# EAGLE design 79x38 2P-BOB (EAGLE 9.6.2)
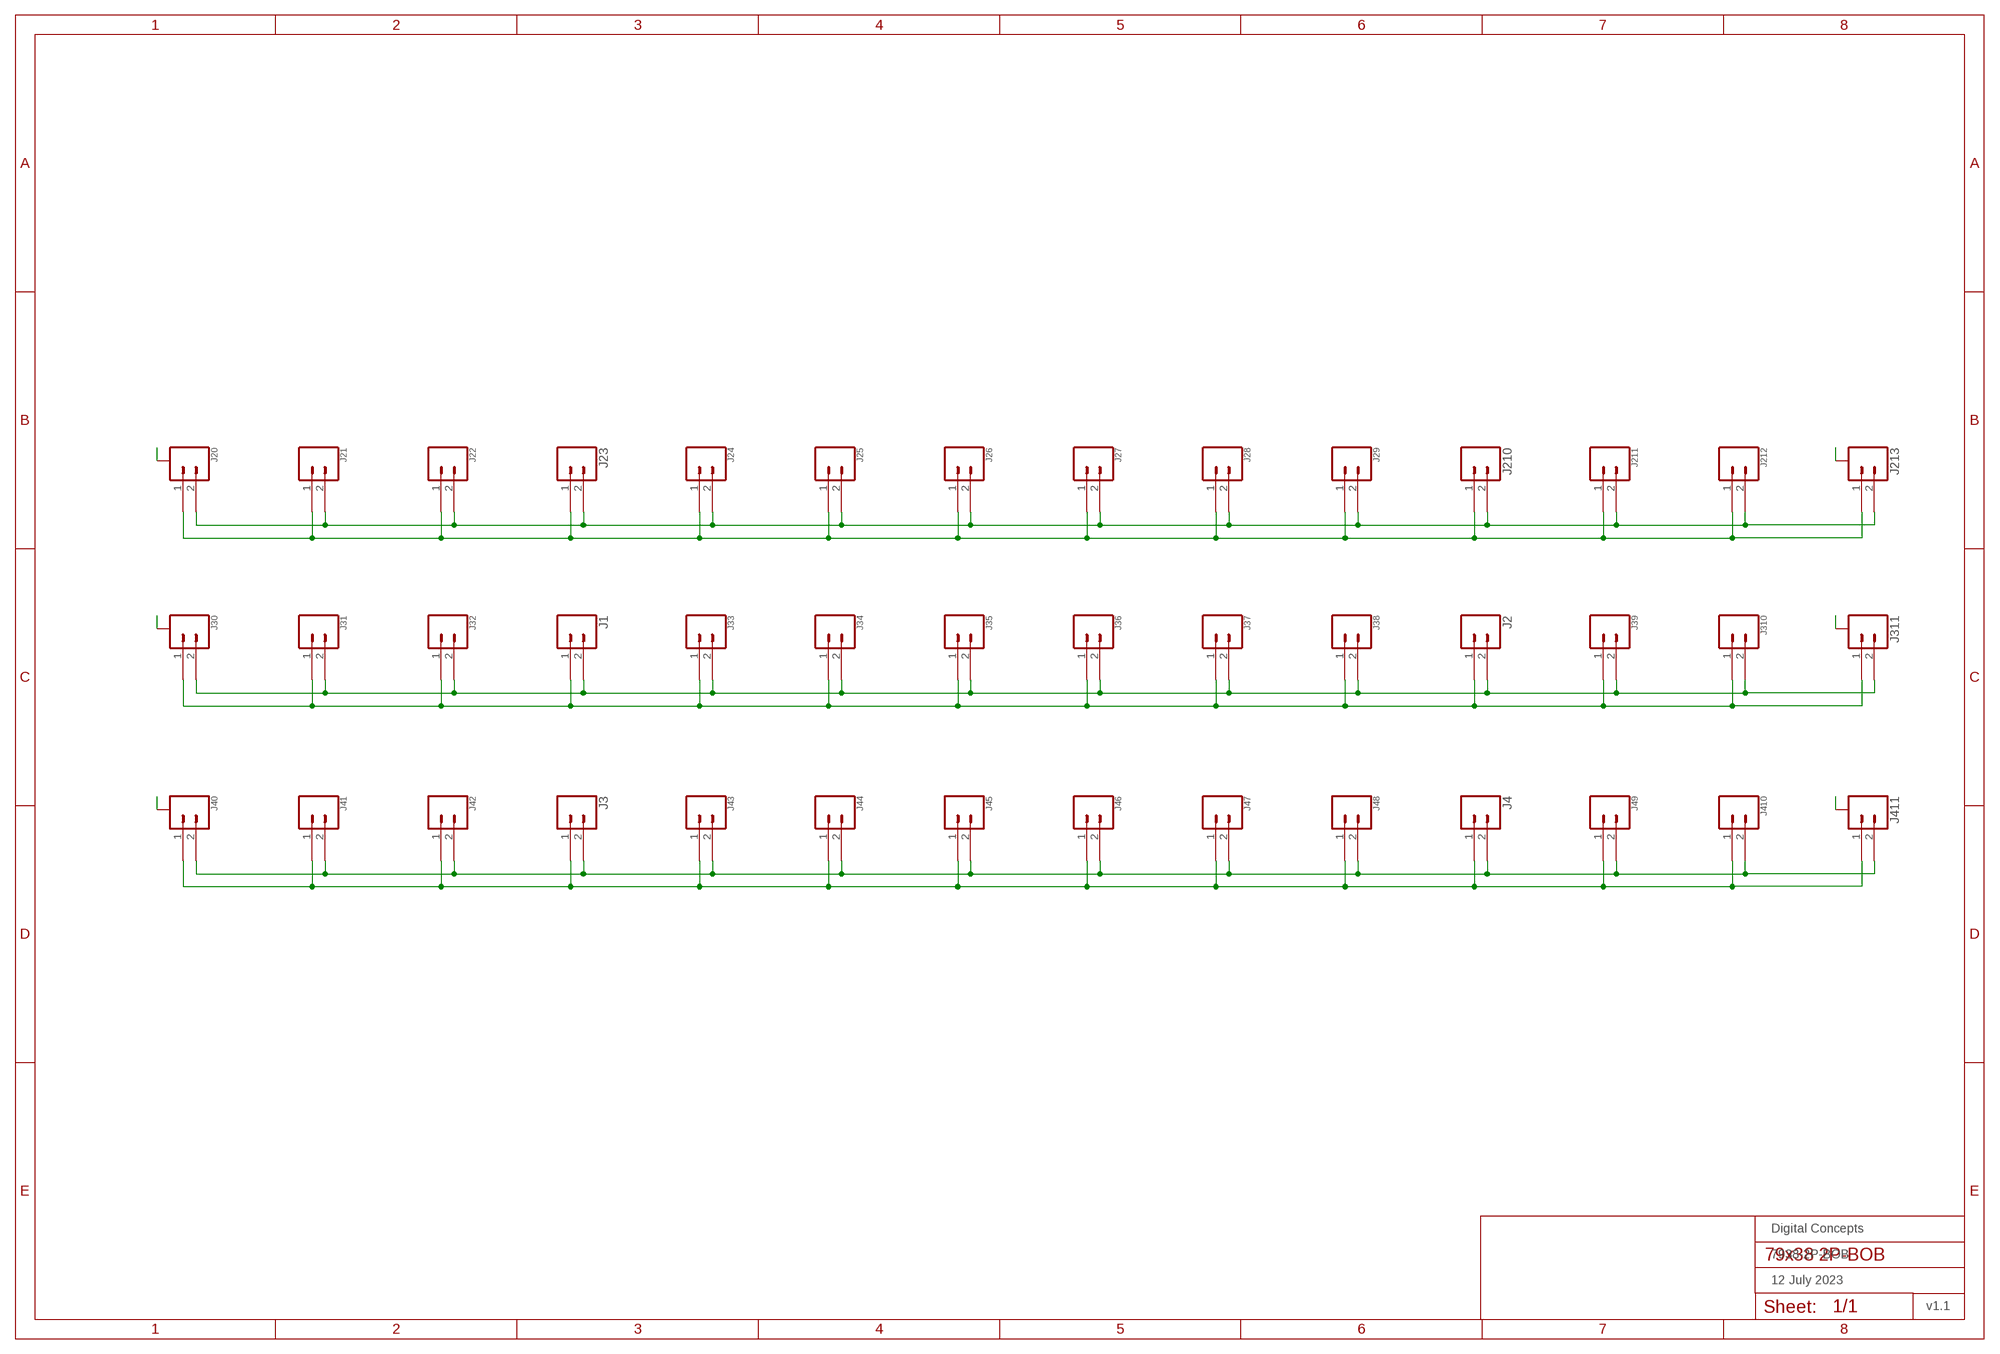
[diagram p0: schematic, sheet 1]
FRAME1 (FRAME-A3L-LOC): DATE: 12 July 2023; OWNER: Digital Concepts; TITLE: 7938-2P-BOB; VERSION: v1.1

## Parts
J1  JST-XH2.54-2-VERTICAL  [JST-XH2.4-2-VERTICAL]
J2  JST-XH2.54-2-VERTICAL  [JST-XH2.4-2-VERTICAL]
J3  JST-XH2.54-2-VERTICAL  [JST-XH2.4-2-VERTICAL]
J4  JST-XH2.54-2-VERTICAL  [JST-XH2.4-2-VERTICAL]
J20  JST-SH1.0-2-SMD-VERTICAL  [JST-SH1.0-2-VERTICAL]
J21  JST-GH1.25-2-VERTICAL  [JST-GH1.25-2-VERTICAL]
J22  JST-PH2.0-2-VERTICAL  [JST-PH2.0-2-VERTICAL]
J23  JST-XH2.54-2-VERTICAL  [JST-XH2.4-2-VERTICAL]
J24  HEADER-1X2-GENERIC  [CONN_02-GENERIC]
J25  HEADER-1X2-GENERIC  [CONN_02-GENERIC]
J26  HEADER-1X2-GENERIC  [CONN_02-GENERIC]
J27  HEADER-1X2-GENERIC  [CONN_02-GENERIC]
J28  HEADER-1X2-GENERIC  [CONN_02-GENERIC]
J29  HEADER-1X2-GENERIC  [CONN_02-GENERIC]
J30  JST-SH1.0-2-SMD-VERTICAL  [JST-SH1.0-2-VERTICAL]
J31  JST-GH1.25-2-VERTICAL  [JST-GH1.25-2-VERTICAL]
J32  JST-PH2.0-2-VERTICAL  [JST-PH2.0-2-VERTICAL]
J33  HEADER-1X2-GENERIC  [CONN_02-GENERIC]
J34  HEADER-1X2-GENERIC  [CONN_02-GENERIC]
J35  HEADER-1X2-GENERIC  [CONN_02-GENERIC]
J36  HEADER-1X2-GENERIC  [CONN_02-GENERIC]
J37  HEADER-1X2-GENERIC  [CONN_02-GENERIC]
J38  HEADER-1X2-GENERIC  [CONN_02-GENERIC]
J39  JST-PH2.0-2-VERTICAL  [JST-PH2.0-2-VERTICAL]
J40  JST-SH1.0-2-SMD-VERTICAL  [JST-SH1.0-2-VERTICAL]
J41  JST-GH1.25-2-VERTICAL  [JST-GH1.25-2-VERTICAL]
J42  JST-PH2.0-2-VERTICAL  [JST-PH2.0-2-VERTICAL]
J43  HEADER-1X2-GENERIC  [CONN_02-GENERIC]
J44  HEADER-1X2-GENERIC  [CONN_02-GENERIC]
J45  HEADER-1X2-GENERIC  [CONN_02-GENERIC]
J46  HEADER-1X2-GENERIC  [CONN_02-GENERIC]
J47  HEADER-1X2-GENERIC  [CONN_02-GENERIC]
J48  HEADER-1X2-GENERIC  [CONN_02-GENERIC]
J49  JST-PH2.0-2-VERTICAL  [JST-PH2.0-2-VERTICAL]
J210  JST-XH2.54-2-VERTICAL  [JST-XH2.4-2-VERTICAL]
J211  JST-PH2.0-2-VERTICAL  [JST-PH2.0-2-VERTICAL]
J212  JST-GH1.25-2-VERTICAL  [JST-GH1.25-2-VERTICAL]
J213  JST-SH1.0-2-SMD-VERTICAL  [JST-SH1.0-2-VERTICAL]
J310  JST-GH1.25-2-VERTICAL  [JST-GH1.25-2-VERTICAL]
J311  JST-SH1.0-2-SMD-VERTICAL  [JST-SH1.0-2-VERTICAL]
J410  JST-GH1.25-2-VERTICAL  [JST-GH1.25-2-VERTICAL]
J411  JST-SH1.0-2-SMD-VERTICAL  [JST-SH1.0-2-VERTICAL]

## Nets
A: J20.A@1(A) J20.A@2(A) J30.A@1(A) J30.A@2(A) J40.A@1(A) J40.A@2(A) J213.A@1(A) J213.A@2(A) J311.A@1(A) J311.A@2(A) J411.A@1(A) J411.A@2(A)
N$1: J20.1 J21.1 J22.1 J23.1 J24.1 J25.1 J26.1 J27.1 J28.1 J29.1 J210.1 J211.1 J212.1 J213.1
N$2: J1.2 J2.2 J30.2 J31.2 J32.2 J33.2 J34.2 J35.2 J36.2 J37.2 J38.2 J39.2 J310.2 J311.2
N$3: J1.1 J2.1 J30.1 J31.1 J32.1 J33.1 J34.1 J35.1 J36.1 J37.1 J38.1 J39.1 J310.1 J311.1
N$4: J3.2 J4.2 J40.2 J41.2 J42.2 J43.2 J44.2 J45.2 J46.2 J47.2 J48.2 J49.2 J410.2 J411.2
N$5: J3.1 J4.1 J40.1 J41.1 J42.1 J43.1 J44.1 J45.1 J46.1 J47.1 J48.1 J49.1 J410.1 J411.1
N$7: J20.2 J21.2 J22.2 J23.2 J24.2 J25.2 J26.2 J27.2 J28.2 J29.2 J210.2 J211.2 J212.2 J213.2

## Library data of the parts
J1-J4 J23 J210 = digitalconcepts:JST-XH2.54-2-VERTICAL: XH2.54 2P Vertical Connector
J20 J30 J40 J213 J311 J411 = digitalconcepts:JST-SH1.0-2-SMD-VERTICAL: JST SH1.0 2P SMD Vertical Connector
J21 J31 J41 J212 J310 J410 = digitalconcepts:JST-GH1.25-2-VERTICAL: JST GH1.25 2P PTH Connector
J22 J32 J39 J42 J49 J211 = digitalconcepts:JST-PH2.0-2-VERTICAL: PH2.0 2P Vertical Connector
J24-J29 J33-J38 J43-J48 = digitalconcepts:HEADER-1X2-GENERIC: Single Row 2-Pin Header

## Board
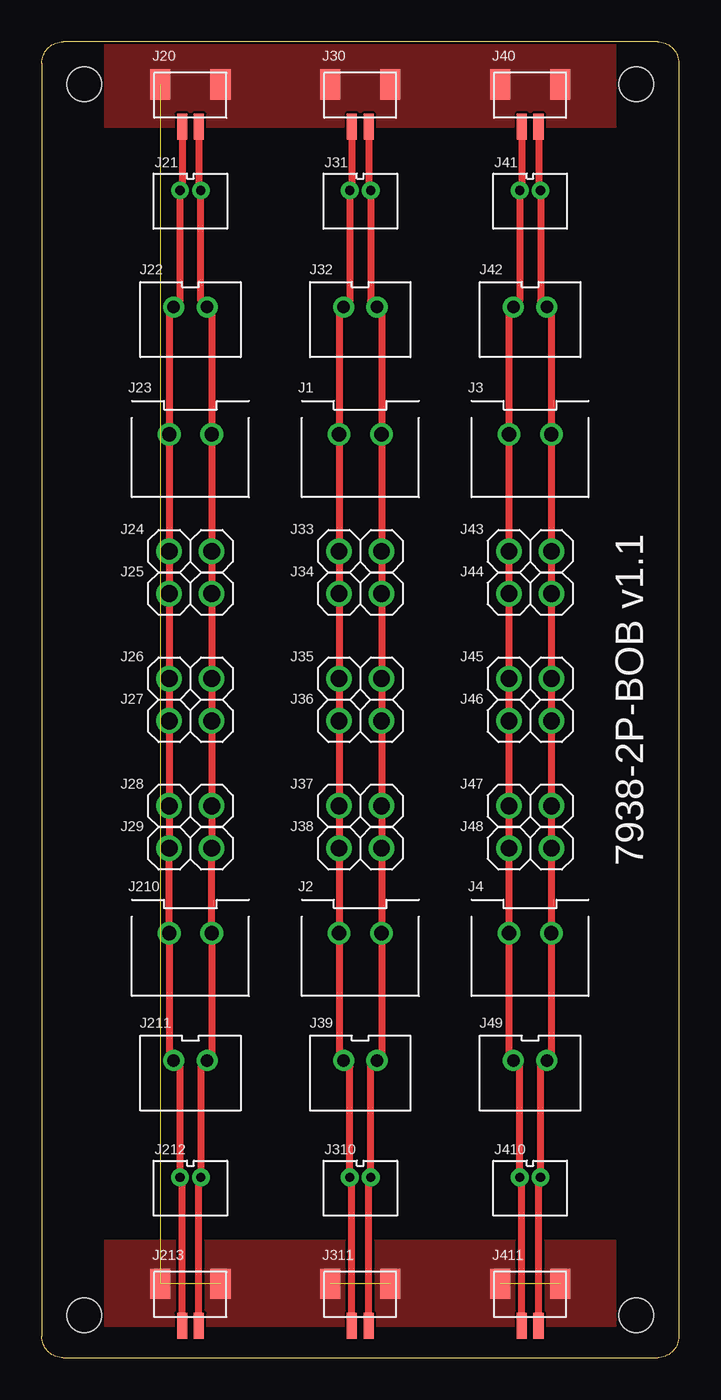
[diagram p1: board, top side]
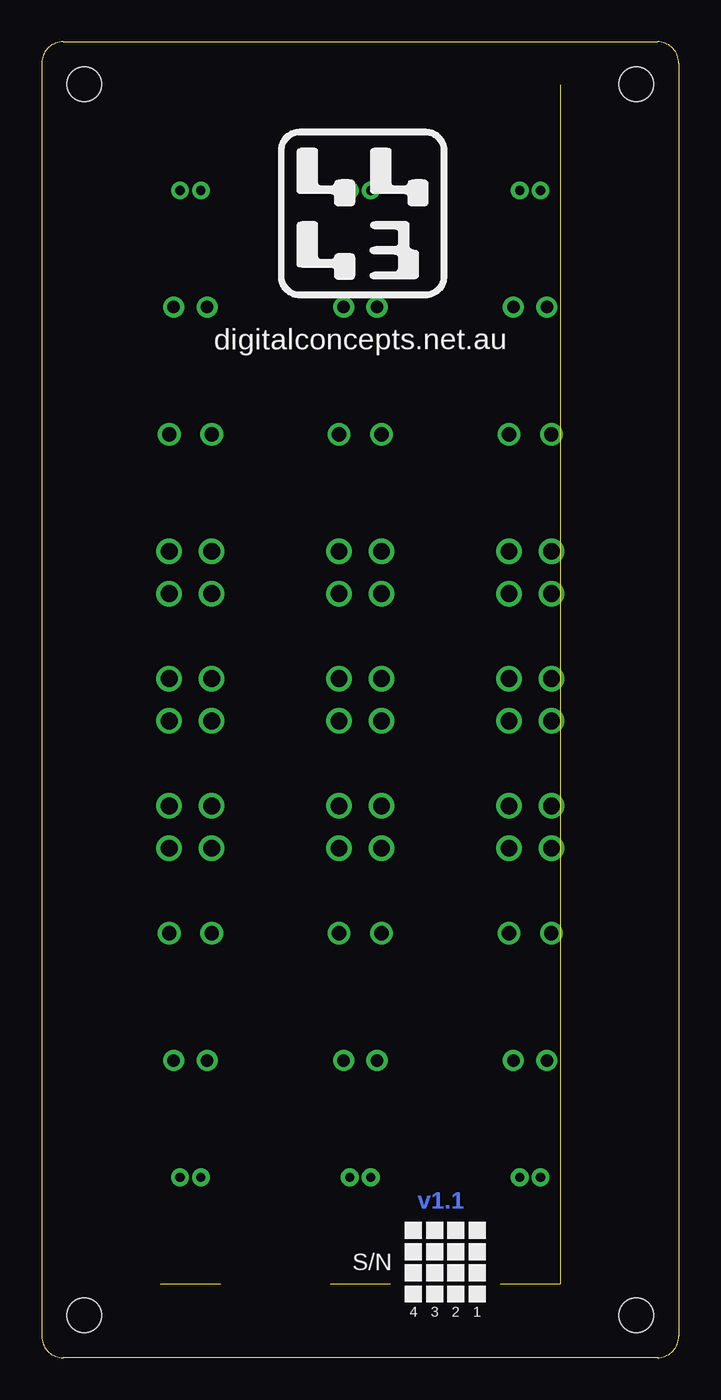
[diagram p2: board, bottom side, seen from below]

Size 38.1 x 78.74 mm. Coordinates in mm from the lower left corner, seen from the top.
Outline: 36.83,78.74 arc-90 38.1,77.47 38.1,1.27 arc-90 36.83,0 1.27,0 arc-90 0,1.27 0,77.47 arc-90 1.27,78.74 36.83,78.74
Copper layers (1*16): Top 0.035mm / dielectric 1.5mm / Bottom 0.035mm
Design rules "default *": minimum track width 6mil, minimum drill 0.35mm, track to track 6mil, track to pad 6mil, pad to pad 6mil, via to via 6mil, smd to smd 6mil, copper to edge 6mil, drill to drill 6mil, minimum pad ring 10mil, minimum via ring 8mil, stop-mask expansion 4mil, vias tented up to drill 0mil, thermal gap 0mil
Holes 2.03 mm at 2.54,76.2 2.54,2.54 35.56,2.54 35.56,76.2

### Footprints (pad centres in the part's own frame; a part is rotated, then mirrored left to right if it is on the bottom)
JST-XH2.4-2-VERTICAL = drill 0.85: 1 -1.27,0; 2 1.27,0
JST-SH1.0-2-VERTICAL = smd 0.6 x 1.55: 1 -0.5,-2.54; 2 0.5,-2.54 | smd 1.2 x 1.8: A@1 -1.8,-0.015; A@2 1.8,-0.015
JST-GH1.25-2-VERTICAL = drill 0.55 pad 1.016: 1 -0.625,0; 2 0.625,0
JST-PH2.0-2-VERTICAL = drill 0.75: 1 -1,0; 2 1,0
CONN_02-GENERIC = drill 1 pad 1.524: 1 0,0; 2 2.54,0

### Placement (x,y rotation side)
J1  19.05,55.24 0 top
J2  19.05,25.4 0 top
J3  29.21,55.24 0 top
J4  29.21,25.4 0 top
J20  8.89,76.2 0 top
J21  8.89,69.85 0 top
J22  8.89,62.87 0 top
J23  8.89,55.24 0 top
J24  7.62,48.26 0 top
J25  7.62,45.72 0 top
J26  7.62,40.64 0 top
J27  7.62,38.1 0 top
J28  7.62,33.02 0 top
J29  7.62,30.48 0 top
J30  19.05,76.2 0 top
J31  19.05,69.85 0 top
J32  19.05,62.87 0 top
J33  17.78,48.26 0 top
J34  17.78,45.72 0 top
J35  17.78,40.64 0 top
J36  17.78,38.1 0 top
J37  17.78,33.02 0 top
J38  17.78,30.48 0 top
J39  19.05,17.78 0 top
J40  29.21,76.2 0 top
J41  29.21,69.85 0 top
J42  29.21,62.87 0 top
J43  27.94,48.26 0 top
J44  27.94,45.72 0 top
J45  27.94,40.64 0 top
J46  27.94,38.1 0 top
J47  27.94,33.02 0 top
J48  27.94,30.48 0 top
J49  29.21,17.78 0 top
J210  8.89,25.4 0 top
J211  8.89,17.78 0 top
J212  8.89,10.79 0 top
J213  8.89,4.45 0 top
J310  19.05,10.79 0 top
J311  19.05,4.45 0 top
J410  29.21,10.79 0 top
J411  29.21,4.45 0 top

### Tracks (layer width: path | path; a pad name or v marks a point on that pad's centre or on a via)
A  (4 unrouted)
  pour Top: 3.81,78.74 34.29,78.74 34.29,73.66 3.81,73.66
  pour Top: 3.81,1.91 34.29,1.91 34.29,6.99 3.81,6.99
N$1
  Top 0.406: J20.1 8.39,69.97 J21.1 8.27,63.24 J22.1 7.62,62.59 J23.1 J24.1 J25.1 J26.1 J27.1 J28.1 J29.1 J210.1 7.62,18.05 J211.1 8.27,17.41 J212.1 8.39,10.67 J213.1
N$2
  Top 0.406: J30.2 19.55,69.97 J31.2 19.68,63.24 J32.2 20.32,62.59 J1.2 J33.2 J34.2 J35.2 J36.2 J37.2 J38.2 J2.2 20.32,18.05 J39.2 19.68,17.41 J310.2 19.55,10.67 J311.2
N$3
  Top 0.406: J30.1 18.55,69.97 J31.1 18.43,63.24 J32.1 17.78,62.59 J1.1 J33.1 J34.1 J35.1 J36.1 J37.1 J38.1 J2.1 17.78,18.05 J39.1 18.43,17.41 J310.1 18.55,10.67 J311.1
N$4
  Top 0.406: J40.2 29.71,69.97 J41.2 29.84,63.24 J42.2 30.48,62.59 J3.2 J43.2 J44.2 J45.2 J46.2 J47.2 J48.2 J4.2 30.48,18.05 J49.2 29.84,17.41 J410.2 29.71,10.67 J411.2
N$5
  Top 0.406: J40.1 28.71,69.97 J41.1 28.59,63.24 J42.1 27.94,62.59 J3.1 J43.1 J44.1 J45.1 J46.1 J47.1 J48.1 J4.1 27.94,18.05 J49.1 28.59,17.41 J410.1 28.71,10.67 J411.1
N$7
  Top 0.406: J20.2 9.39,69.97 J21.2 9.52,63.24 J22.2 10.16,62.59 J23.2 J24.2 J25.2 J26.2 J27.2 J28.2 J29.2 J210.2 10.16,18.05 J211.2 9.52,17.41 J212.2 9.39,10.67 J213.2

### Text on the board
Bottom: v1.1
tPlace: 7938-2P-BOB v1.1
bPlace: digitalconcepts.net.au | S/N | 1 | 2 | 3 | 4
